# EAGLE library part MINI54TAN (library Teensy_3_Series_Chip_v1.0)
MINI54TAN Bootloader from PJRC.com, preprogrammed with Teensy 3.0 bootloader. https://www.pjrc.com/store/ic_mini54_tqfp.html
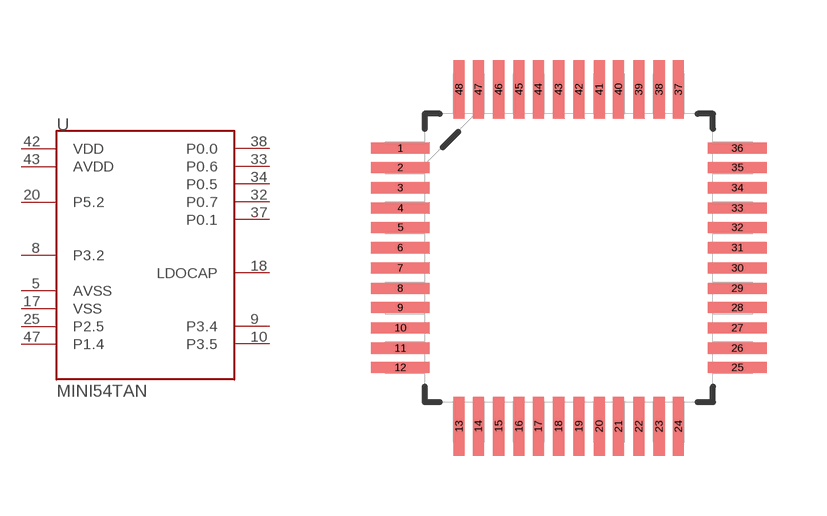
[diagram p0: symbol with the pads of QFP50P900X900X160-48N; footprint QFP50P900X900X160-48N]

Designator prefix -

## MINI54TANDEFAULT  [QFP50P900X900X160-48N]
5  AVSS
8  P3.2
9  P3.4
10  P3.5
17  VSS
18  LDOCAP
20  P5.2
25  P2.5
32  P0.7
33  P0.6
34  P0.5
37  P0.1
38  P0.0
42  VDD
43  AVDD
47  P1.4

## Footprint QFP50P900X900X160-48N (pad centres in mm)
smd 1.473 x 0.279: 1 -4.216,2.743; 2 -4.216,2.261; 3 -4.216,1.753; 4 -4.216,1.245; 5 -4.216,0.762; 6 -4.216,0.254; 7 -4.216,-0.254; 8 -4.216,-0.762; 9 -4.216,-1.245; 10 -4.216,-1.753; 11 -4.216,-2.261; 12 -4.216,-2.743; 25 4.216,-2.743; 26 4.216,-2.261; 27 4.216,-1.753; 28 4.216,-1.245; 29 4.216,-0.762; 30 4.216,-0.254; 31 4.216,0.254; 32 4.216,0.762; 33 4.216,1.245; 34 4.216,1.753; 35 4.216,2.261; 36 4.216,2.743
smd 0.279 x 1.473: 13 -2.743,-4.216; 14 -2.261,-4.216; 15 -1.753,-4.216; 16 -1.245,-4.216; 17 -0.762,-4.216; 18 -0.254,-4.216; 19 0.254,-4.216; 20 0.762,-4.216; 21 1.245,-4.216; 22 1.753,-4.216; 23 2.261,-4.216; 24 2.743,-4.216; 37 2.743,4.216; 38 2.261,4.216; 39 1.753,4.216; 40 1.245,4.216; 41 0.762,4.216; 42 0.254,4.216; 43 -0.254,4.216; 44 -0.762,4.216; 45 -1.245,4.216; 46 -1.753,4.216; 47 -2.261,4.216; 48 -2.743,4.216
